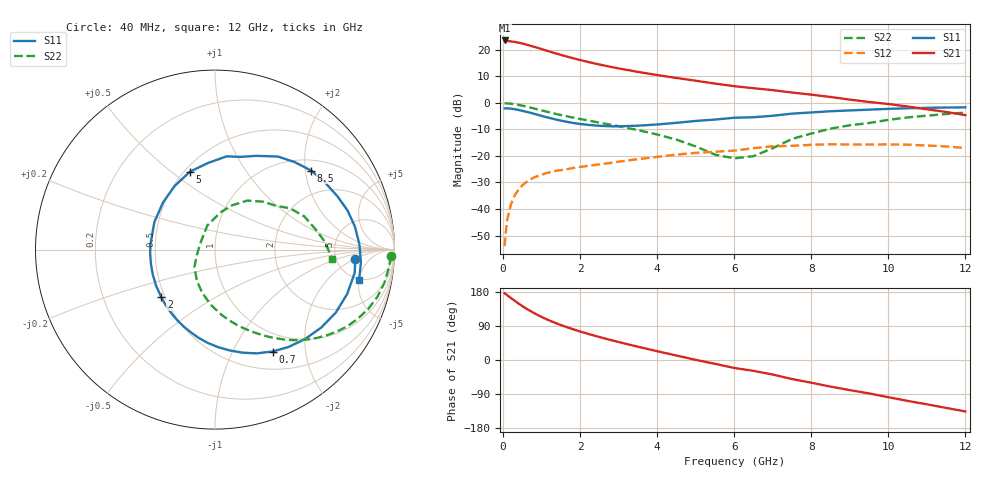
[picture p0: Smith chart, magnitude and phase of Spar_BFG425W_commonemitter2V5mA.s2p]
! Filename: 25bfg425.001
! BFG425W Field C1
! V1=8.298E-001V,V2=2.000E+000V, I1=6.614E-005A, I2=5.000E-003A
# GHz  S  MA  R 50
!  S11  S21  S12  S22
!Freq(GHz)  Mag  Ang  Mag  Ang  Mag  Ang  Mag  Ang
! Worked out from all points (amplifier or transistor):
!   44 points, 40 MHz to 12 GHz, reference 50 ohm
!   highest |S21| = 23.5 dB at 40 MHz (marker M1)
!   |S21| within 3 dB of that: start of sweep to 944.9 MHz
!   unconditionally stable (mu >= 1): 2.439 GHz to end of sweep
!   at 700 MHz: K = 0.33, MSG = 25.2 dB, |S12| = -28.9 dB
!   at 2.4 GHz: K = 0.99, MSG = 19.1 dB, |S12| = -23.3 dB
!   at 12 GHz: K = 1.49, MAG = 2.0 dB, |S12| = -17.0 dB
!   S11 on the Smith chart (normalised r, x): 40 MHz: 7.64, -2.08; 700 MHz: 0.73, -1.45; 2 GHz: 0.48, -0.30; 5 GHz: 0.53, +0.58; 8.5 GHz: 1.27, +2.15; 12 GHz: 4.77, -5.02
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0.04  0.783 -3.9  14.94 176.1  0.002 76.6  0.979 -2.1
0.1  0.789 -9.3  14.62 171.6  0.006 85.0  0.976 -5.5
0.2  0.777 -18.6  14.36 163.8  0.012 78.7  0.962 -11.0
0.4  0.734 -36.3  13.59 149.2  0.023 69.0  0.915 -21.3
0.5  0.707 -44.8  13.11 142.1  0.028 64.6  0.884 -25.8
0.7  0.652 -60.6  11.93 129.8  0.036 56.7  0.817 -34.1
0.8  0.623 -68.1  11.37 124.0  0.039 53.5  0.783 -37.6
1  0.567 -81.9  10.28 113.6  0.044 48.0  0.72 -44.0
1.3  0.5 -100.5  8.816 100.2  0.051 41.7  0.637 -52.0
1.6  0.447 -117.8  7.635 88.6  0.056 37.2  0.569 -58.5
2  0.4 -138.4  6.395 75.2  0.062 32.8  0.497 -66.3
2.2  0.385 -148.3  5.899 69.2  0.065 31.0  0.466 -70.0
2.6  0.366 -167.0  5.083 57.9  0.071 27.6  0.411 -77.3
3  0.361 175.5  4.445 47.4  0.078 24.2  0.363 -84.7
3.5  0.371 155.6  3.825 35.1  0.087 19.6  0.307 -94.7
4.5  0.42 122.2  2.941 11.9  0.106 8.5  0.203 -119.6
5  0.456 107.8  2.607 0.4  0.114 1.3  0.151 -139.4
6  0.524 82.8  2.058 -21.1  0.126 -12.6  0.09 150.5
6.5  0.535 74.9  1.884 -28.7  0.14 -14.1  0.099 132.6
8.5  0.694 39.4  1.289 -70.2  0.166 -49.4  0.327 56.6
10.5  0.79 9.3  0.853 -107.9  0.163 -84.0  0.531 20.4
12  0.821 -12.1  0.586 -135.8  0.141 -114.1  0.655 -4.6
